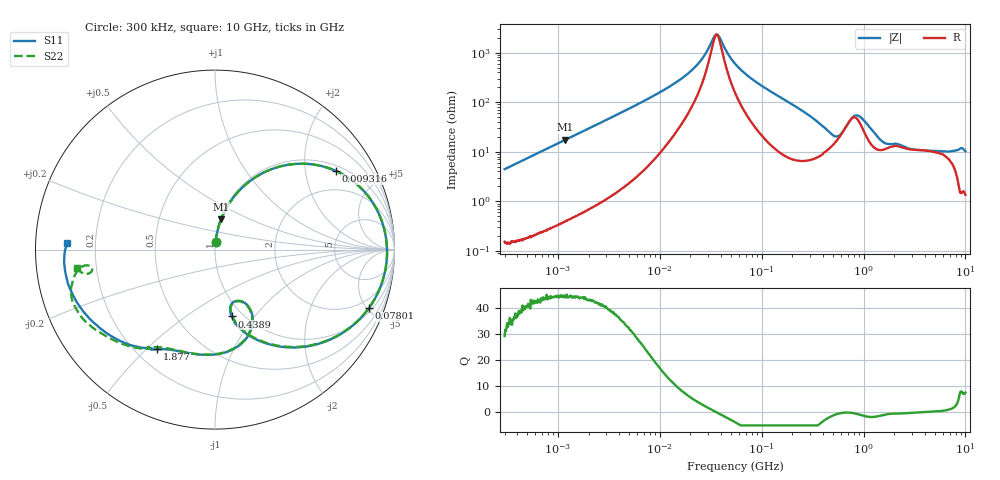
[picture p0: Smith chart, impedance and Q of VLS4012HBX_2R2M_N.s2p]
! S-Parameter Data Generated by TDK Corporation
! Copyright(C) 2023 TDK Corporation.
! All Rights Reserved.
! TDK P/N: VLS4012HBX-2R2M-N (Inductor)
! Property: L=2.2uH at 1MHz
! Size(LxWxT): 4x4x1.2mm
! Model Type: s2p (Touchstone File Format Version 1.0)
! Frequency: DC=Yes Start=0.3MHz Stop=10000MHz 802points Log-sweep
! Model Generated on June 16, 2023
! Port Assignments:
!  1 ---@@@--- 2
! Applicable Conditions:
!  Temperature = 25 degC
!  DC Bias Current = 0 A
!  Small Signal Operation
! Terms and conditions regarding TDK Simulation Models
! (1)This simulation model is being provided solely for informational purposes. Please refer to the specifications of the products in terms of detailed characteristics of such products.
! (2)In no event shall TDK Corporation of any of its subsidiaries be liable for any loss or damage arising, directly or indirectly,
!  From any information contained in this simulation model, including, but not limited to loss or damages arising from any inaccuracies, omissions or errors in connection with such information.
! (3)Any and all copyrights on this simulation model are owned by TDK Corporation.
!  Duplication or redistribution of this simulation model without prior written permission from TDK Corporation is prohibited.
! (4)This simulation model is subject to any modification or change without any prior notice.
! (5)Neither TDK Corporation nor any of its subsidiaries shall make any warranty, express or implied,
!  Including but not limited to the correctness, implied warranties of merchantability and fitness for a particular purpose with respect to this simulation models.
! (6)The use of this simulation model shall be deemed to have consented to the terms and conditions hereof.
# Hz S MA R 50
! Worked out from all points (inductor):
!   801 points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, 300 kHz to 10 GHz, reference 50 ohm
!   read as one part in series: L = 2.36 uH near 318.3 kHz
!   highest Q = 44.5 at 1.187 MHz (marker M1), where L = 2.34 uH
!   self-resonance near 36.21 MHz
!   S11 on the Smith chart (normalised r, x): 300 kHz: 1.00, +0.09; 9.316 MHz: 1.19, +2.93; 78.01 MHz: 1.25, -5.12; 438.9 MHz: 0.89, -0.77; 1.877 GHz: 0.29, -0.54; 10 GHz: 0.10, +0.02
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300000  0.04406 85.5  0.9974 -2.6  0.9976 -2.6  0.04381 85.4
1187016  0.1711 78.8  0.9814 -9.9  0.9813 -9.9  0.1711 78.8
1713600  0.2424 74.6  0.9647 -14.1  0.9647 -14.1  0.2423 74.6
3732762  0.4756 59.9  0.8668 -28.6  0.867 -28.6  0.4757 59.9
9315664  0.8034 33.1  0.5531 -53.8  0.5532 -53.8  0.8035 33.1
9671944  0.8138 31.9  0.5365 -54.8  0.5365 -54.8  0.814 31.9
2.15778e7  0.942 9.9  0.1954 -68.4  0.1955 -68.4  0.9422 10.0
3.598933e7  0.9588 -1.7  0.04116 -4.7  0.04117 -4.7  0.959 -1.6
5.477226e7  0.9478 -11.5  0.1571 63.6  0.1571 63.6  0.948 -11.4
7.800823e7  0.9168 -20.9  0.2948 61.5  0.2948 61.5  0.9172 -20.7
1.653189e8  0.7473 -46.1  0.6138 40.1  0.6138 40.1  0.7475 -45.7
3.126428e8  0.5097 -68.8  0.8041 15.1  0.8042 15.1  0.5103 -68.3
4.388767e8  0.3837 -76.0  0.8329 0.8  0.833 0.8  0.3855 -75.5
6.15965e8  0.3099 -67.1  0.7696 -15.4  0.7697 -15.4  0.3131 -67.0
8.18524e8  0.476 -64.3  0.5993 -18.6  0.5993 -18.6  0.4789 -65.1
1.24442e9  0.5921 -100.2  0.6924 -21.6  0.6925 -21.6  0.5917 -101.9
1.767019e9  0.6258 -117.5  0.6493 -39.9  0.6493 -39.9  0.6263 -119.7
1.876852e9  0.6413 -120.0  0.6284 -42.9  0.6285 -42.9  0.6407 -122.1
4.399376e9  0.8119 -155.2  0.3759 -76.8  0.3759 -76.8  0.8194 -149.6
6.899057e9  0.8423 -169.7  0.2837 -94.9  0.2837 -95.0  0.8388 -162.8
8.322921e9  0.8397 -177.8  0.2435 -106.2  0.2436 -106.2  0.7445 -172.7
1e10  0.826 177.6  0.2315 -111.0  0.2315 -111.0  0.7767 -172.6
